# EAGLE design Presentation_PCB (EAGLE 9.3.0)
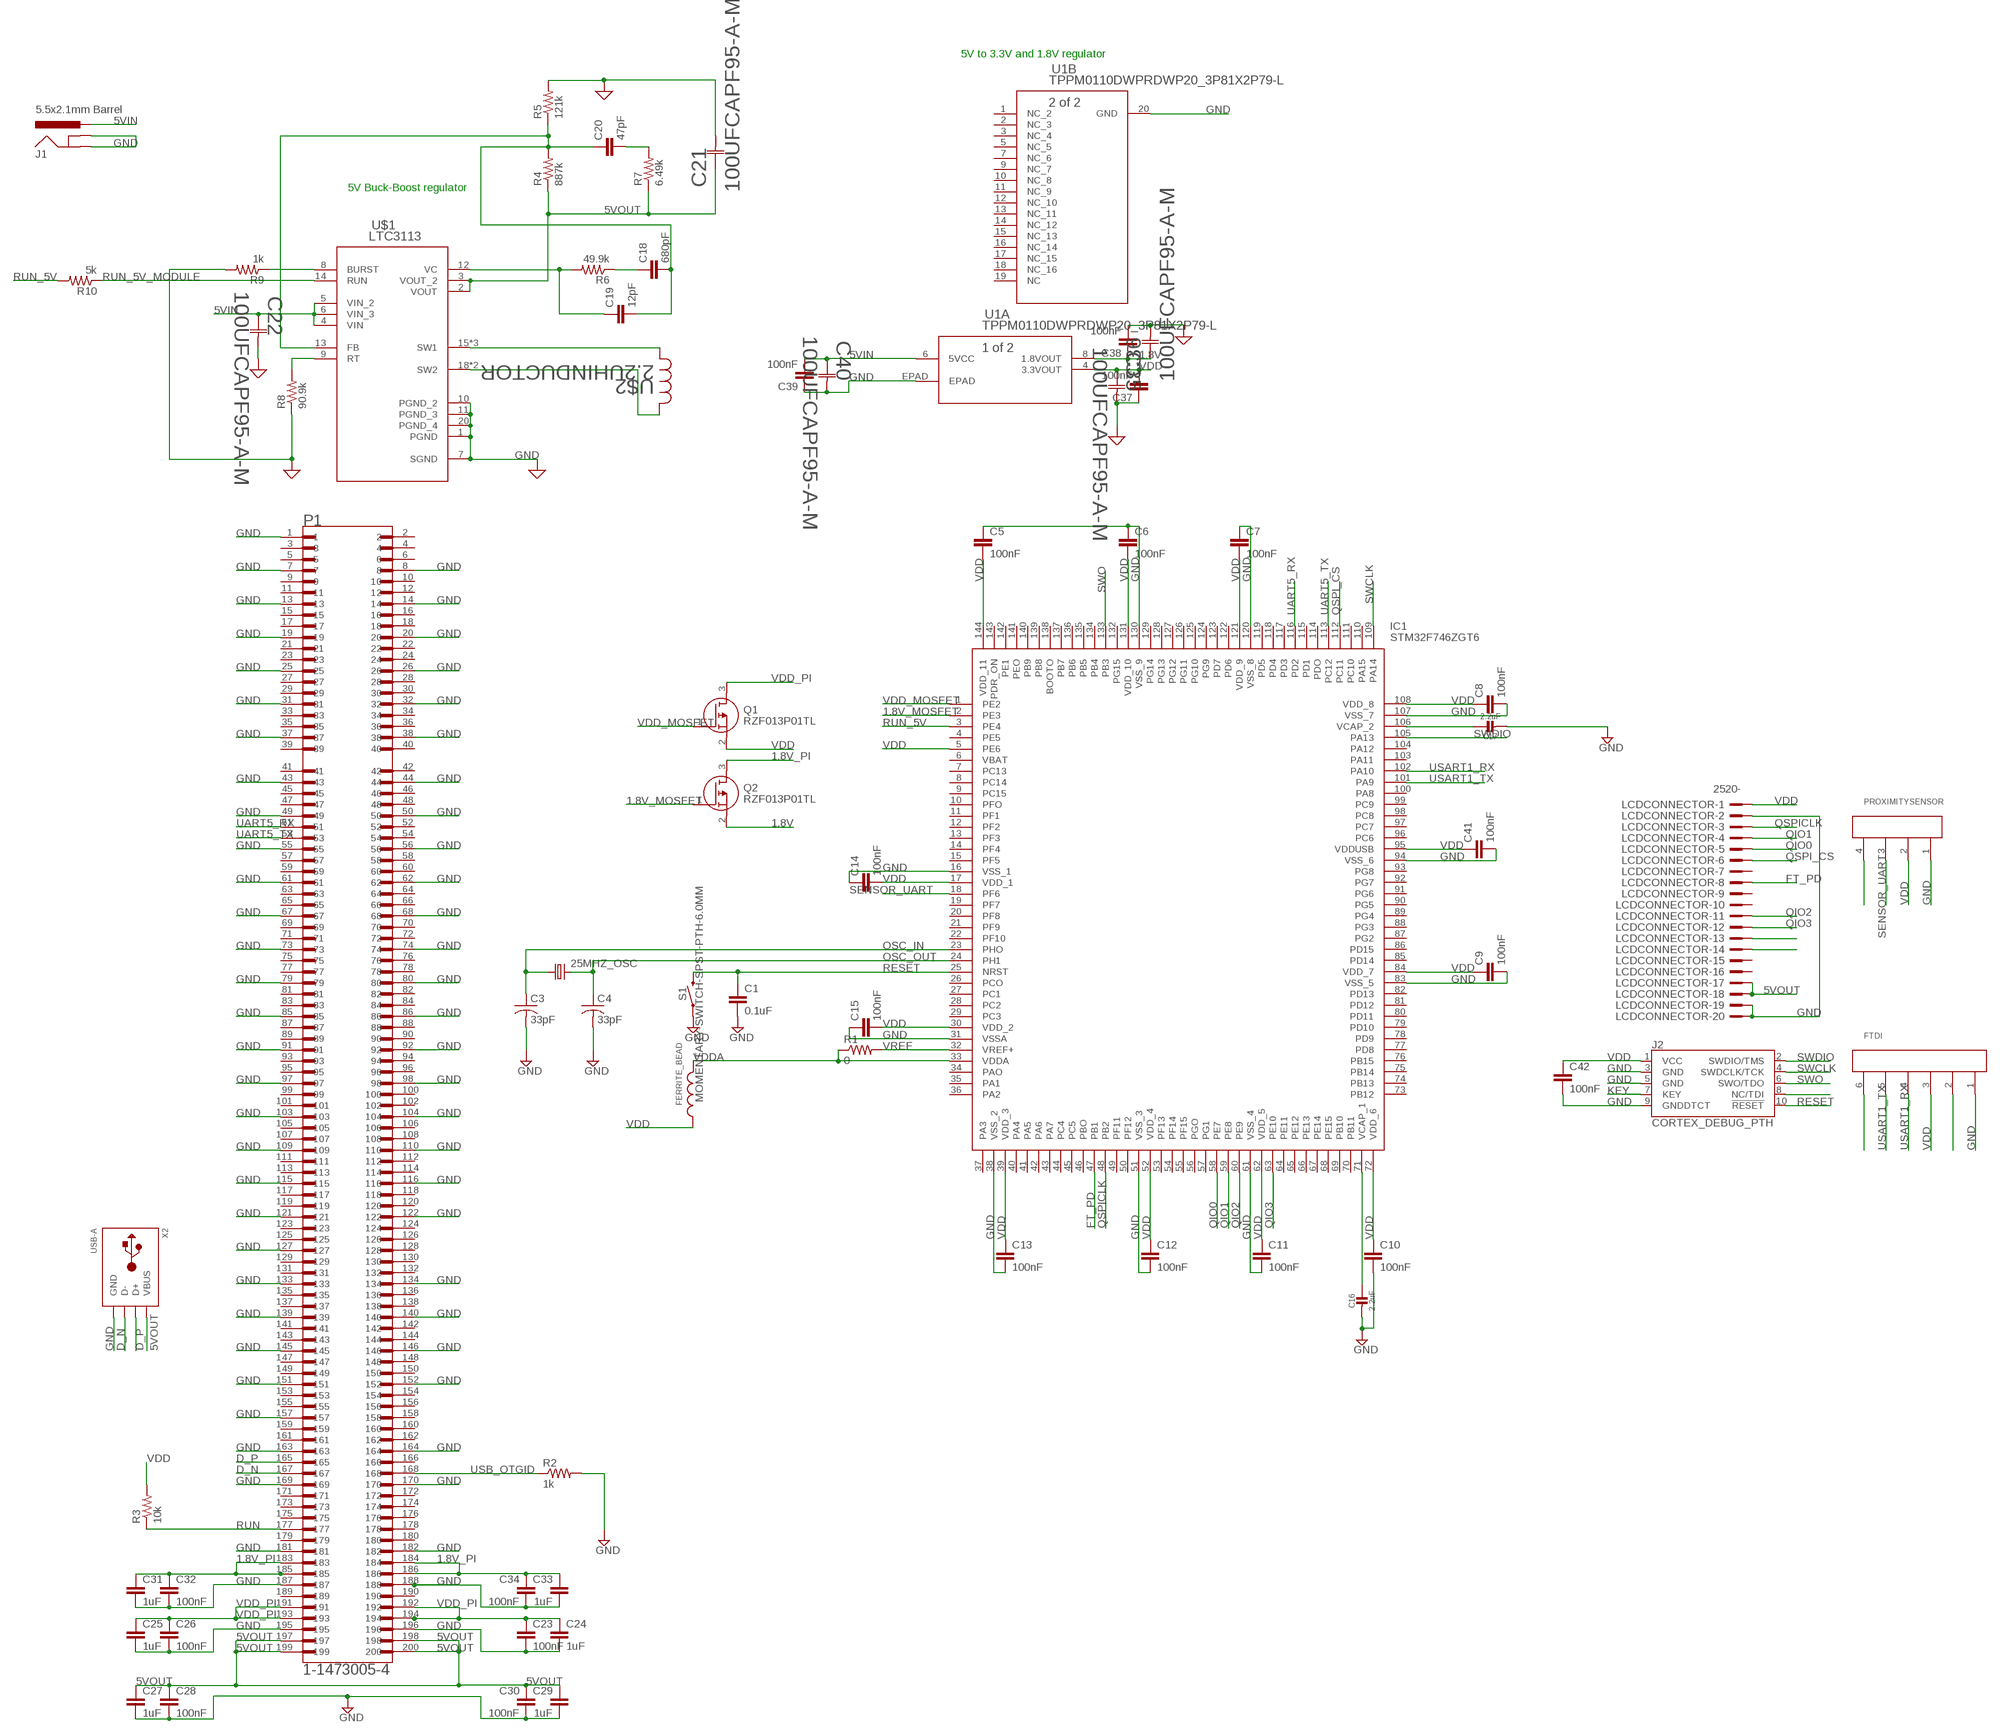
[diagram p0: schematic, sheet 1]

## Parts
25MHZ_OSC  CRYSTALHC49UP  [HC49UP]
C1  0.1uF  C-EUC0805  [C0805]
C3  33pF  C-USC0805  [C0805]
C4  33pF  C-USC0805  [C0805]
C5  100nF  C-EUC0805  [C0805]
C6  100nF  C-EUC0805  [C0805]
C7  100nF  C-EUC0805  [C0805]
C8  100nF  C-EUC0805  [C0805]
C9  100nF  C-EUC0805  [C0805]
C10  100nF  C-EUC0805  [C0805]
C11  100nF  C-EUC0805  [C0805]
C12  100nF  C-EUC0805  [C0805]
C13  100nF  C-EUC0805  [C0805]
C14  100nF  C-EUC0805  [C0805]
C15  100nF  C-EUC0805  [C0805]
C16  2.2uF  CAP_CERAMIC0805-NOOUTLINE  [0805-NO]
C17  2.2uF  CAP_CERAMIC0805-NOOUTLINE  [0805-NO]
C18  680pF  C-EUC0805  [C0805]
C19  12pF  C-EUC0805  [C0805]
C20  47pF  C-EUC0805  [C0805]
C21  100UFCAPF95-A-M  [F95-A-M]
C22  100UFCAPF95-A-M  [F95-A-M]
C23  100nF  C-EUC0805  [C0805]
C24  1uF  C-EUC0805  [C0805]
C25  1uF  C-EUC0805  [C0805]
C26  100nF  C-EUC0805  [C0805]
C27  1uF  C-EUC0805  [C0805]
C28  100nF  C-EUC0805  [C0805]
C29  1uF  C-EUC0805  [C0805]
C30  100nF  C-EUC0805  [C0805]
C31  1uF  C-EUC0805  [C0805]
C32  100nF  C-EUC0805  [C0805]
C33  1uF  C-EUC0805  [C0805]
C34  100nF  C-EUC0805  [C0805]
C35  100UFCAPF95-A-M  [F95-A-M]
C36  100UFCAPF95-A-M  [F95-A-M]
C37  100nF  C-EUC0805  [C0805]
C38  100nF  C-EUC0805  [C0805]
C39  100nF  C-EUC0805  [C0805]
C40  100UFCAPF95-A-M  [F95-A-M]
C41  100nF  C-EUC0805  [C0805]
C42  100nF  C-EUC0805  [C0805]
FERRITE_BEAD  WE-CBA_0805_782853112_HC  [WE-CBA_0805(W=4)]
FTDI  66100611622  [66100611622]
IC1  STM32F746ZGT6  [QFP50P2200X2200X160-144N]
J1  5.5x2.1mm Barrel  POWER_JACKSMD  [POWER_JACK_SMD]
J2  CORTEX_DEBUG_PTH  [2X5-PTH-1.27MM]
LCDCONNECTOR  2520-  [PAK100/2500-20]
P1  1-1473005-4  [TE_1-1473005-4]
PROXIMITYSENSOR  66100411622  [66100411622]
Q1  RZF013P01TL  [SOT65P210X85-3N]
Q2  RZF013P01TL  [SOT65P210X85-3N]
R1  0  R-US_R0805  [R0805]
R2  1k  R-US_R0805  [R0805]
R3  10k  R-US_R0805  [R0805]
R4  887k  R-US_R0805  [R0805]
R5  121k  R-US_R0805  [R0805]
R6  49.9k  R-US_R0805  [R0805]
R7  6.49k  R-US_R0805  [R0805]
R8  90.9k  R-US_R0805  [R0805]
R9  1k  R-US_R0805  [R0805]
R10  5k  R-US_R0805  [R0805]
S1  MOMENTARY-SWITCH-SPST-PTH-6.0MM  [TACTILE_SWITCH_PTH_6.0MM]
U1  TPPM0110DWPRDWP20_3P81X2P79-L  [DWP20_3P81X2P79-L]
U$1  LTC3113  [TSSOP-20_FE/CA]
U$2  2.2UHINDUCTOR  [IND_10040]
X2  USB-A  [MOLEX_480371000]

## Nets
1.8V: C36.1 C38.1 Q2.2(S) U1.8(A:1.8VOUT)
1.8V_MOSFET: IC1.2(PE3) Q2.1(G)
1.8V_PI: C31.1 C32.1 C33.1 C34.1 P1.183 P1.184 P1.185 P1.186 Q2.3(D)
5VIN: C22.1 C39.2 C40.1 J1.VIN0(PWR) U1.6(A:5VCC) U$1.4(VIN) U$1.5(VIN_2) U$1.6(VIN_3)
5VOUT: C21.1 C27.1 C28.1 C29.1 C30.1 LCDCONNECTOR.17 LCDCONNECTOR.18 P1.197 P1.198 P1.199 P1.200 R4.1 R7.1 U$1.2(VOUT) U$1.3(VOUT_2) X2.1(VBUS)
D_N [D]: P1.167 X2.2(D-)
D_P [D]: P1.165 X2.3(D+)
FT_PD: IC1.47(PB1) LCDCONNECTOR.8
GND: C1.2 C3.2 C4.2 C5.1 C6.1 C7.1 C8.2 C9.2 C10.2 C11.2 C12.2 C13.2 C14.1 C15.1 C16.2 C17.2 C21.2 C22.2 C23.2 C24.2 C25.2 C26.2 C27.2 C28.2 C29.2 C30.2 C31.2 C32.2 C33.2 C34.2 C35.2 C36.2 C37.1 C38.2 C39.1 C40.2 C41.2 C42.2 FTDI.1 IC1.16(VSS_1) IC1.31(VSSA) IC1.38(VSS_2) IC1.51(VSS_3) IC1.61(VSS_4) IC1.83(VSS_5) IC1.94(VSS_6) IC1.107(VSS_7) IC1.120(VSS_8) IC1.130(VSS_9) J1.GND(GNDBREAK) J1.P$4(GND) J2.3(GND) J2.5(GND) J2.9(GNDDTCT) LCDCONNECTOR.2 LCDCONNECTOR.19 LCDCONNECTOR.20 P1.1 P1.7 P1.8 P1.13 P1.14 P1.19 P1.20 P1.25 P1.26 P1.31 P1.32 P1.37 P1.38 P1.43 P1.44 P1.49 P1.50 P1.55 P1.56 P1.61 P1.62 P1.67 P1.68 P1.73 P1.74 P1.79 P1.80 P1.85 P1.86 P1.91 P1.92 P1.97 P1.98 P1.103 P1.104 P1.109 P1.110 P1.115 P1.116 P1.121 P1.122 P1.127 P1.133 P1.134 P1.139 P1.140 P1.145 P1.146 P1.151 P1.152 P1.157 P1.163 P1.164 P1.169 P1.170 P1.181 P1.182 P1.187 P1.188 P1.195 P1.196 PROXIMITYSENSOR.1 R2.2 R5.2 R8.1 R9.2 S1.1 U1.20(B:GND) U1.EPAD(A:EPAD) U$1.1(PGND) U$1.7(SGND) U$1.10(PGND_2) U$1.11(PGND_3) U$1.20(PGND_4) X2.4(GND) ; supply symbol labelled SUP
KEY: J2.7(KEY)
N$1: C16.1 IC1.71(VCAP_1)
N$2: C17.1 IC1.106(VCAP_2)
N$3: C20.2 R7.2
N$4: C19.1 R6.2 U$1.12(VC)
N$5: C18.1 R6.1
N$6: C18.2 C19.2 C20.1 R4.2 R5.1 U$1.13(FB)
N$7: U$1.15(SW1) U$1.16(SW1) U$1.17(SW1) U$2.2
N$8: U$1.18(SW2) U$1.19(SW2) U$2.1
N$9: R8.2 U$1.9(RT)
N$10: R9.1 U$1.8(BURST)
N$12: FTDI.2
N$15: PROXIMITYSENSOR.4
N$16: FTDI.6
N$19: J2.8(NC/TDI)
N$20: LCDCONNECTOR.13
N$21: LCDCONNECTOR.14
OSC_IN: 25MHZ_OSC.1 C3.1 IC1.23(PHO)
OSC_OUT: 25MHZ_OSC.2 C4.1 IC1.24(PH1)
QIO0: IC1.58(PE7) LCDCONNECTOR.5
QIO1: IC1.59(PE8) LCDCONNECTOR.4
QIO2: IC1.60(PE9) LCDCONNECTOR.11
QIO3: IC1.63(PE10) LCDCONNECTOR.12
QSPI_CS: IC1.112(PC11) LCDCONNECTOR.6
QSPICLK: IC1.48(PB2) LCDCONNECTOR.3
RESET: C1.1 IC1.25(NRST) J2.10(!RESET) S1.3
RUN: P1.177 R3.1
RUN_5V: IC1.3(PE4) R10.2
RUN_5V_MODULE: R10.1 U$1.14(RUN)
SENSOR_UART: IC1.18(PF6) PROXIMITYSENSOR.3
SWCLK: IC1.109(PA14) J2.4(SWDCLK/TCK)
SWDIO: IC1.105(PA13) J2.2(SWDIO/TMS)
SWO: IC1.133(PB3) J2.6(SWO/TDO)
UART5_RX: IC1.116(PD2) P1.51
UART5_TX: IC1.113(PC12) P1.53
USART1_RX: FTDI.4 IC1.102(PA10)
USART1_TX: FTDI.5 IC1.101(PA9)
USB_OTGID: P1.168 R2.1
VDD: C5.2 C6.2 C7.2 C8.1 C9.1 C10.1 C11.1 C12.1 C13.1 C14.2 C15.2 C35.1 C37.2 C41.1 C42.1 FERRITE_BEAD.1 FTDI.3 IC1.5(PE6) IC1.17(VDD_1) IC1.30(VDD_2) IC1.39(VDD_3) IC1.52(VDD_4) IC1.62(VDD_5) IC1.72(VDD_6) IC1.84(VDD_7) IC1.95(VDDUSB) IC1.108(VDD_8) IC1.121(VDD_9) IC1.131(VDD_10) IC1.144(VDD_11) J2.1(VCC) LCDCONNECTOR.1 PROXIMITYSENSOR.2 Q1.2(S) R3.2 U1.4(A:3.3VOUT)
VDD_MOSFET: IC1.1(PE2) Q1.1(G)
VDD_PI: C23.1 C24.1 C25.1 C26.1 P1.191 P1.192 P1.193 P1.194 Q1.3(D)
VDDA: FERRITE_BEAD.2 IC1.33(VDDA) R1.1
VREF: IC1.32(VREF+) R1.2
Unconnected: IC1.4(PE5) IC1.6(VBAT) IC1.7(PC13) IC1.8(PC14) IC1.9(PC15) IC1.10(PFO) IC1.11(PF1) IC1.12(PF2) IC1.13(PF3) IC1.14(PF4) IC1.15(PF5) IC1.19(PF7) IC1.20(PF8) IC1.21(PF9) IC1.22(PF10) IC1.26(PCO) IC1.27(PC1) IC1.28(PC2) IC1.29(PC3) IC1.34(PAO) IC1.35(PA1) IC1.36(PA2) IC1.37(PA3) IC1.40(PA4) IC1.41(PA5) IC1.42(PA6) IC1.43(PA7) IC1.44(PC4) IC1.45(PC5) IC1.46(PBO) IC1.49(PF11) IC1.50(PF12) IC1.53(PF13) IC1.54(PF14) IC1.55(PF15) IC1.56(PGO) IC1.57(PG1) IC1.64(PE11) IC1.65(PE12) IC1.66(PE13) IC1.67(PE14) IC1.68(PE15) IC1.69(PB10) IC1.70(PB11) IC1.73(PB12) IC1.74(PB13) IC1.75(PB14) IC1.76(PB15) IC1.77(PD8) IC1.78(PD9) IC1.79(PD10) IC1.80(PD11) IC1.81(PD12) IC1.82(PD13) IC1.85(PD14) IC1.86(PD15) IC1.87(PG2) IC1.88(PG3) IC1.89(PG4) IC1.90(PG5) IC1.91(PG6) IC1.92(PG7) IC1.93(PG8) IC1.96(PC6) IC1.97(PC7) IC1.98(PC8) IC1.99(PC9) IC1.100(PA8) IC1.103(PA11) IC1.104(PA12) IC1.110(PA15) IC1.111(PC10) IC1.114(PDO) IC1.115(PD1) IC1.117(PD3) IC1.118(PD4) IC1.119(PD5) IC1.122(PD6) IC1.123(PD7) IC1.124(PG9) IC1.125(PG10) IC1.126(PG11) IC1.127(PG12) IC1.128(PG13) IC1.129(PG14) IC1.132(PG15) IC1.134(PB4) IC1.135(PB5) IC1.136(PB6) IC1.137(PB7) IC1.138(BOOTO) IC1.139(PB8) IC1.140(PB9) IC1.141(PEO) IC1.142(PE1) IC1.143(PDR_ON) LCDCONNECTOR.7 LCDCONNECTOR.9 LCDCONNECTOR.10 LCDCONNECTOR.15 LCDCONNECTOR.16 P1.2 P1.3 P1.4 P1.5 P1.6 P1.9 P1.10 P1.11 P1.12 P1.15 P1.16 P1.17 P1.18 P1.21 P1.22 P1.23 P1.24 P1.27 P1.28 P1.29 P1.30 P1.33 P1.34 P1.35 P1.36 P1.39 P1.40 P1.41 P1.42 P1.45 P1.46 P1.47 P1.48 P1.52 P1.54 P1.57 P1.58 P1.59 P1.60 P1.63 P1.64 P1.65 P1.66 P1.69 P1.70 P1.71 P1.72 P1.75 P1.76 P1.77 P1.78 P1.81 P1.82 P1.83 P1.84 P1.87 P1.88 P1.89 P1.90 P1.93 P1.94 P1.95 P1.96 P1.99 P1.100 P1.101 P1.102 P1.105 P1.106 P1.107 P1.108 P1.111 P1.112 P1.113 P1.114 P1.117 P1.118 P1.119 P1.120 P1.123 P1.124 P1.125 P1.126 P1.128 P1.129 P1.130 P1.131 P1.132 P1.135 P1.136 P1.137 P1.138 P1.141 P1.142 P1.143 P1.144 P1.147 P1.148 P1.149 P1.150 P1.153 P1.154 P1.155 P1.156 P1.158 P1.159 P1.160 P1.161 P1.162 P1.166 P1.171 P1.172 P1.173 P1.174 P1.175 P1.176 P1.178 P1.179 P1.180 P1.189 P1.190 U1.1(B:NC_2) U1.2(B:NC_3) U1.3(B:NC_4) U1.5(B:NC_5) U1.7(B:NC_6) U1.9(B:NC_7) U1.10(B:NC_8) U1.11(B:NC_9) U1.12(B:NC_10) U1.13(B:NC_11) U1.14(B:NC_12) U1.15(B:NC_13) U1.16(B:NC_14) U1.17(B:NC_15) U1.18(B:NC_16) U1.19(B:NC)

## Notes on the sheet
- 5V to 3.3V and 1.8V regulator
- 5V Buck-Boost regulator

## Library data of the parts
25MHZ_OSC = adafruit:CRYSTAL: CRYSTAL; OC_FARNELL: unknown; OC_NEWARK: unknown
C1 C5-C15 C18-C20 C23-C34 C37-C39 C41 C42 = rcl:C-EU: CAPACITOR, European symbol; SPICEPREFIX: C
C3 C4 = adafruit:C-US: CAPACITOR, American symbol
C16 C17 = audio amplifier example:CAP_CERAMIC
C21 C22 C35 C36 C40 = 477_LIBRARY:100UFCAP; MANUFACTURER_PART_NUMBER: F951A107KAAAQ2; VENDOR: AVX Corporation
FERRITE_BEAD = Wurth_Elektronik_Passive_rev18f:WE-CBA_0805: WE-CBA SMD EMI Suppression Ferrite Bead
FTDI = Wurth_Elektronik_Electromechanic_Wire_to_Board_Connectors_rev18a:66100611622: WIRE TO BOARD CONNECTION - 2.54 MM - SHROUDED HEADER - STRAIGHT - GLOW WIRE PLASTIC - WR-WTB =>ConWTB254 661006116222 Characteristics INSULATOR: PA46G15 FLAMMABILITY RATING: UL94V0 COLOR: BLACK METAL: PHOSPHOR BRONZE PLATING: TIN OVER Ni QUALITY CLASS: 25 MATING CYCLES OPERATING TEMPERATURE:-40°C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
IC1 = 477_LIBRARY:STM32F746ZGT6: ARM Microcontrollers - MCU High-performance and DSP with FPU, ARM Cortex-M7 MCU with 1 Mbytes Flash, 200 MHz CPU, Art Accelerator, L1 cache, SDRAM Source: Datasheet; DESCRIPTION: ARM Microcontrollers - MCU High-performance and DSP with FPU, ARM Cortex-M7 MCU with 1 Mbytes Flash, 200 MHz CPU, Art Accelerator, L1 cache, SDRAM; HEIGHT: 1.6mm; MANUFACTURER_NAME: STMicroelectronics; MANUFACTURER_PART_NUMBER: STM32F746ZGT6; MOUSER_PART_NUMBER: 511-STM32F746ZGT6; MOUSER_PRICE-STOCK: https://www.mouser.com/Search/Refine.aspx?Keyword=511-STM32F746ZGT6; RS_PART_NUMBER: 8820290; RS_PRICE-STOCK: http://uk.rs-online.com/web/p/products/8820290
J1 = SparkFun-Connectors:POWER_JACK: Power Jack Connector This is the standard 5.5mm barrel jack for power. The PTH is the most common, proven, reliable, footprint. The Slot footprint only works if the mill layer is transmitted to the PCB fab house so be warned. Here are the connectors we sell at SparkFun: DC Barrel Power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; PROD_ID: CONN-08106; SF_ID: PRT-12748
J2 = SparkFun-Connectors:CORTEX_DEBUG: Cortex Debug Connector - 10 pin Supports JTAG debug, Serial Wire debug, and Serial Wire Viewer. PTH and SMD connector options available. General Connector Information Products: PTH Connector -via Digi-Key SparkFun PSoc SparkFun T
LCDCONNECTOR = con-3m:2520-: 3M (TM) Pak 100 4-Wall Header Source: 3M; OC_FARNELL: unknown; OC_NEWARK: unknown
P1 = Rpi-DDR2:1-1473005-4: Conn SO DIMM Socket SKT 200 POS 0.6mm Solder RA SMD Tray; AVAILABILITY: Unavailable; CENTERLINE_PITCH: .6 mm[.024 in]; COMMENT: 1-1473005-4; DESCRIPTION: SEMI-HARD TRAY DDR2 SODIMM SOCKET 200P 5; MF: TE Connectivity; MP: 1-1473005-4; NUMBER_OF_POSITIONS: 200; PACKAGE: None; PRICE: None; PRODUCT_TYPE: Socket; TE_PURCHASE_URL: https://www.te.com/usa-en/product-1-1473005-4.html?te_bu=Cor&te_type=disp&te_campaign=seda_glo_cor-seda-global-disp-prtnr-fy19-seda-model-bom-cta_sma-317_1&elqCampaignId=32493
PROXIMITYSENSOR = Wurth_Elektronik_Electromechanic_Wire_to_Board_Connectors_rev18a:66100411622: WIRE TO BOARD CONNECTION - 2.54 MM - SHROUDED HEADER - STRAIGHT - GLOW WIRE PLASTIC - WR-WTB =>ConWTB254 661004116222 Characteristics INSULATOR: PA46G15 FLAMMABILITY RATING: UL94V0 COLOR: BLACK METAL: PHOSPHOR BRONZE PLATING: TIN OVER Ni QUALITY CLASS: 25 MATING CYCLES OPERATING TEMPERATURE:-40°C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
Q1 Q2 = Pchannel:RZF013P01TL: 1.5V Drive Pch MOSFET: MOSFETs are made as ultra-low ON-resistance by the micro-processing technologies suitable for mobilr equipment for low current consumption. In wide lineup including compact type, high-power type and complex type to meet in the market. Source: Datasheet; DESCRIPTION: 1.5V Drive Pch MOSFET: MOSFETs are made as ultra-low ON-resistance by the micro-processing technologies suitable for mobilr equipment for low current consumption. In wide lineup including compact type, high-power type and complex type to meet in the market.; HEIGHT: 0.85mm; MANUFACTURER_NAME: ROHM Semiconductor; MANUFACTURER_PART_NUMBER: RZF013P01TL; MOUSER_PART_NUMBER: 755-RZF013P01TL; MOUSER_PRICE-STOCK: https://www.mouser.com/Search/Refine.aspx?Keyword=755-RZF013P01TL
R1-R3 = audio amplifier example:R-US_: RESISTOR, American symbol
R4-R10 = resistor:R-US_: RESISTOR, American symbol
S1 = SparkFun-Switches:MOMENTARY-SWITCH-SPST: Momentary Switch (Pushbutton) - SPST; PROD_ID: SWCH-08441; SF_SKU: COM-00097
U1 = 477_LIBRARY:TPPM0110DWPR; MANUFACTURER_PART_NUMBER: TPPM0110DWPR; VENDOR: Texas Instruments
U$1 = 477_LIBRARY:LTC3113
U$2 = 477_LIBRARY:2.2UHINDUCTOR
X2 = adafruit:USB-A: USB type A 'plug' Used for things that can directly connect to a USB port, say USB key

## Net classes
1 D: width 0.203 mm

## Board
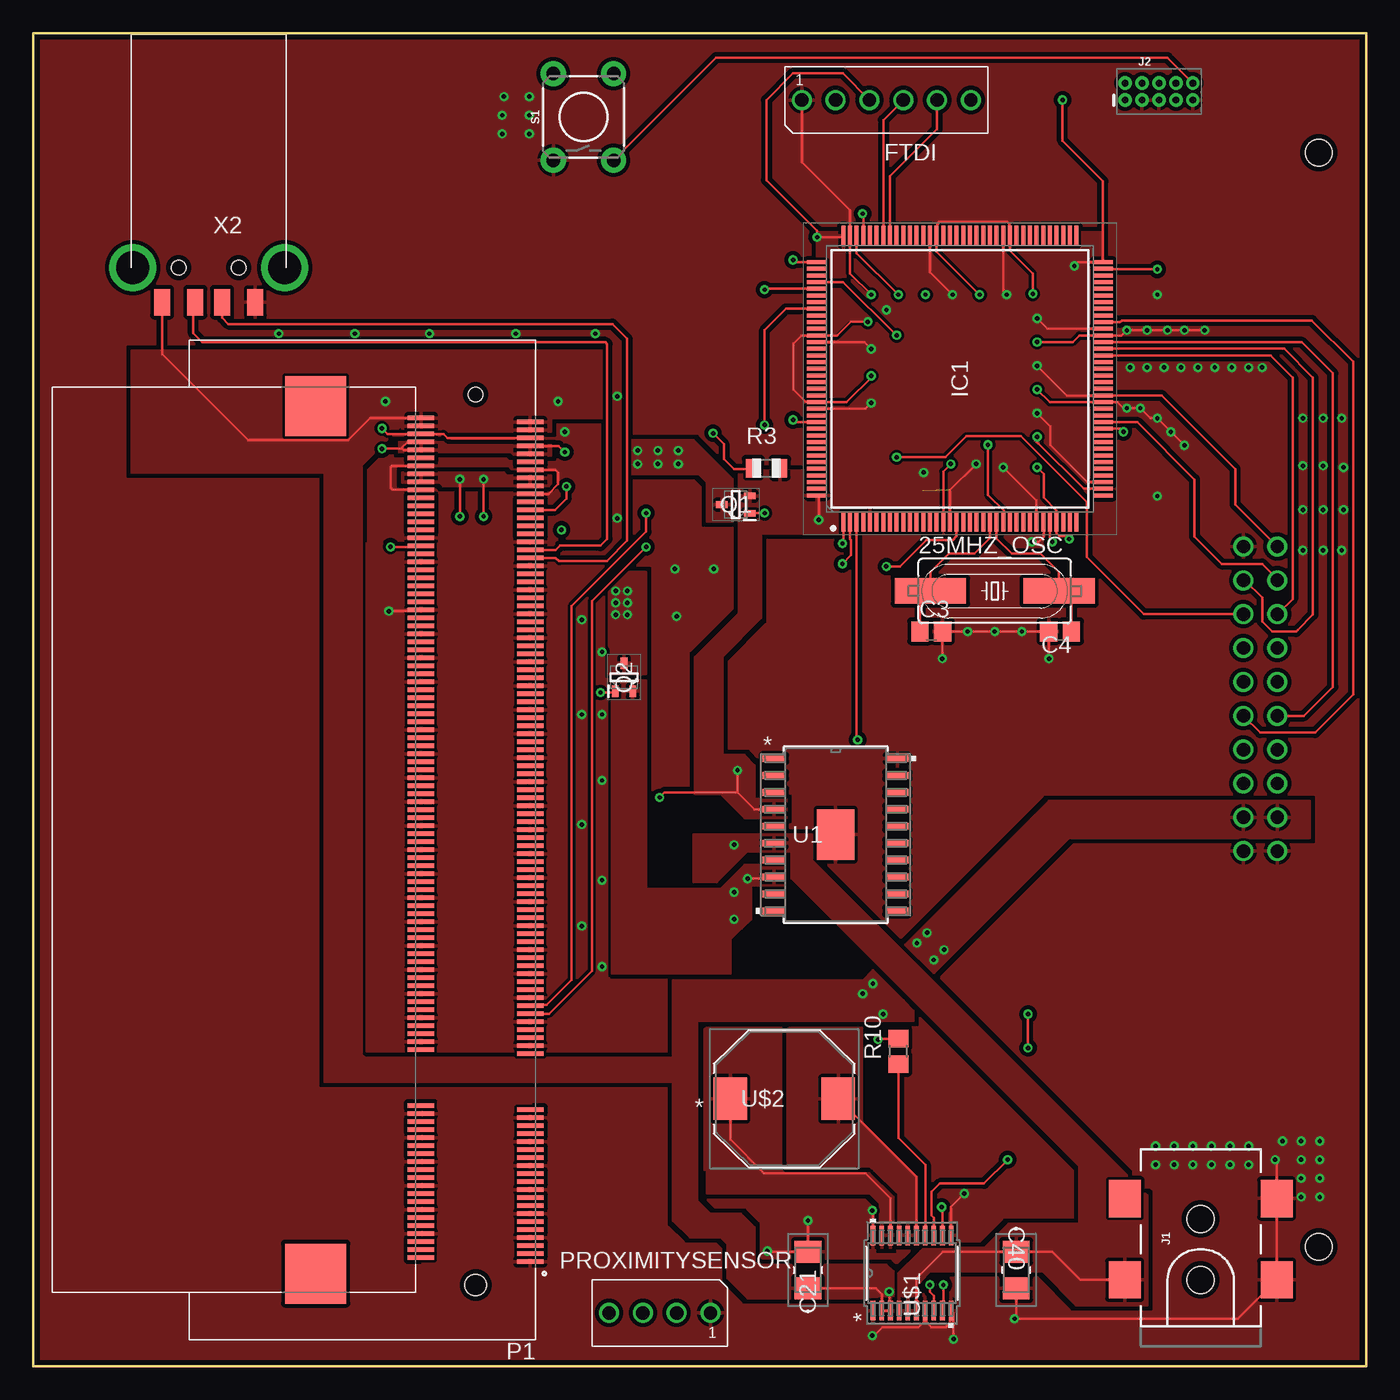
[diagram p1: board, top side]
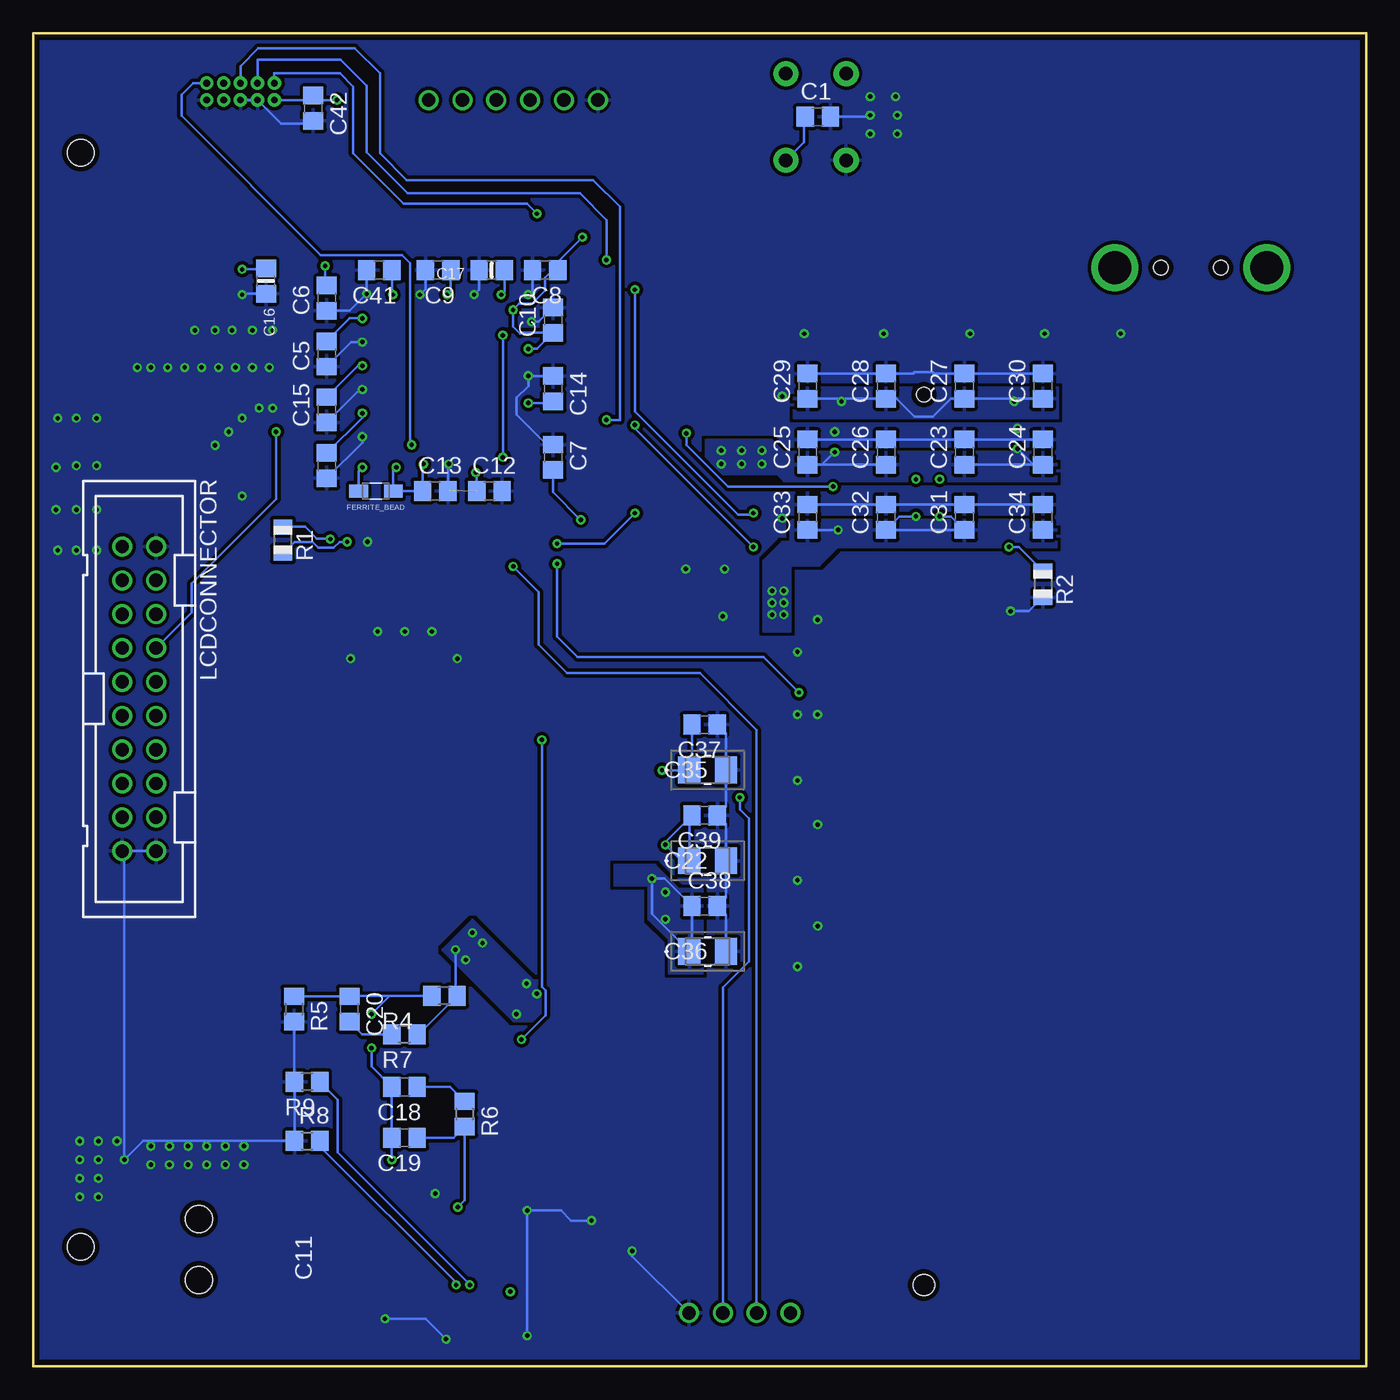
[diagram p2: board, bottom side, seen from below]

Size 100 x 100 mm. Coordinates in mm from the lower left corner, seen from the top.
Outline: 0,0 100,0 100,100 0,100 0,0
Copper layers (1*16): Top 0.0356mm / dielectric 1.5011mm / Bottom 0.0356mm
Design rules "ECE_Senior_Design": minimum track width 8mil, minimum drill 13mil, track to track 8mil, track to pad 8mil, pad to pad 6mil, via to via 8mil, smd to smd 6mil, copper to edge 15mil, drill to drill 8mil, minimum pad ring 7mil, minimum via ring 7mil, stop-mask expansion 3mil, vias tented up to drill 0mil, thermal gap 10mil
Holes 2 mm at 96.45,8.95 96.45,91.05

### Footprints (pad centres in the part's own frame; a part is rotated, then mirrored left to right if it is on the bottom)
HC49UP = smd 5.334 x 1.93: 1 -4.826,0; 2 4.826,0
C0805 = smd 1.3 x 1.5: 1 -0.95,0; 2 0.95,0
C0805' = smd 1.3 x 1.5: 1 -0.85,0; 2 0.85,0
0805-NO = smd 1.3 x 1.5: 1 -0.95,0; 2 0.95,0
F95-A-M = smd 1.651 x 2.007: 1 -1.384,0; 2 1.384,0
WE-CBA_0805(W=4) = smd 1.4 x 1: 1 -1.3,0; 2 1.3,0
66100611622 = drill 1: 1 6.35,0; 2 3.81,0; 3 1.27,0; 4 -1.27,0; 5 -3.81,0; 6 -6.35,0
QFP50P2200X2200X160-144N = smd 1.475 x 0.3: 1 -10.738,8.75; 2 -10.738,8.25; 3 -10.738,7.75; 4 -10.738,7.25; 5 -10.738,6.75; 6 -10.738,6.25; 7 -10.738,5.75; 8 -10.738,5.25; 9 -10.738,4.75; 10 -10.738,4.25; 11 -10.738,3.75; 12 -10.738,3.25; 13 -10.738,2.75; 14 -10.738,2.25; 15 -10.738,1.75; 16 -10.738,1.25; 17 -10.738,0.75; 18 -10.738,0.25; 19 -10.738,-0.25; 20 -10.738,-0.75; 21 -10.738,-1.25; 22 -10.738,-1.75; 23 -10.738,-2.25; 24 -10.738,-2.75; 25 -10.738,-3.25; 26 -10.738,-3.75; 27 -10.738,-4.25; 28 -10.738,-4.75; 29 -10.738,-5.25; 30 -10.738,-5.75; 31 -10.738,-6.25; 32 -10.738,-6.75; 33 -10.738,-7.25; 34 -10.738,-7.75; 35 -10.738,-8.25; 36 -10.738,-8.75; 73 10.738,-8.75; 74 10.738,-8.25; 75 10.738,-7.75; 76 10.738,-7.25; 77 10.738,-6.75; 78 10.738,-6.25; 79 10.738,-5.75; 80 10.738,-5.25; 81 10.738,-4.75; 82 10.738,-4.25; 83 10.738,-3.75; 84 10.738,-3.25; 85 10.738,-2.75; 86 10.738,-2.25; 87 10.738,-1.75; 88 10.738,-1.25; 89 10.738,-0.75; 90 10.738,-0.25; 91 10.738,0.25; 92 10.738,0.75; 93 10.738,1.25; 94 10.738,1.75; 95 10.738,2.25; 96 10.738,2.75; 97 10.738,3.25; 98 10.738,3.75; 99 10.738,4.25; 100 10.738,4.75; 101 10.738,5.25; 102 10.738,5.75; 103 10.738,6.25; 104 10.738,6.75; 105 10.738,7.25; 106 10.738,7.75; 107 10.738,8.25; 108 10.738,8.75 | smd 0.3 x 1.475: 37 -8.75,-10.738; 38 -8.25,-10.738; 39 -7.75,-10.738; 40 -7.25,-10.738; 41 -6.75,-10.738; 42 -6.25,-10.738; 43 -5.75,-10.738; 44 -5.25,-10.738; 45 -4.75,-10.738; 46 -4.25,-10.738; 47 -3.75,-10.738; 48 -3.25,-10.738; 49 -2.75,-10.738; 50 -2.25,-10.738; 51 -1.75,-10.738; 52 -1.25,-10.738; 53 -0.75,-10.738; 54 -0.25,-10.738; 55 0.25,-10.738; 56 0.75,-10.738; 57 1.25,-10.738; 58 1.75,-10.738; 59 2.25,-10.738; 60 2.75,-10.738; 61 3.25,-10.738; 62 3.75,-10.738; 63 4.25,-10.738; 64 4.75,-10.738; 65 5.25,-10.738; 66 5.75,-10.738; 67 6.25,-10.738; 68 6.75,-10.738; 69 7.25,-10.738; 70 7.75,-10.738; 71 8.25,-10.738; 72 8.75,-10.738; 109 8.75,10.738; 110 8.25,10.738; 111 7.75,10.738; 112 7.25,10.738; 113 6.75,10.738; 114 6.25,10.738; 115 5.75,10.738; 116 5.25,10.738; 117 4.75,10.738; 118 4.25,10.738; 119 3.75,10.738; 120 3.25,10.738; 121 2.75,10.738; 122 2.25,10.738; 123 1.75,10.738; 124 1.25,10.738; 125 0.75,10.738; 126 0.25,10.738; 127 -0.25,10.738; 128 -0.75,10.738; 129 -1.25,10.738; 130 -1.75,10.738; 131 -2.25,10.738; 132 -2.75,10.738; 133 -3.25,10.738; 134 -3.75,10.738; 135 -4.25,10.738; 136 -4.75,10.738; 137 -5.25,10.738; 138 -5.75,10.738; 139 -6.25,10.738; 140 -6.75,10.738; 141 -7.25,10.738; 142 -7.75,10.738; 143 -8.25,10.738; 144 -8.75,10.738
POWER_JACK_SMD = smd 2.8 x 2.4: GND 0,-5.7; P$4 6.1,-5.7; VIN0 0,5.7; VIN1 6.1,5.7 | hole 2.032: 0,0; 4.572,0
2X5-PTH-1.27MM = drill 0.508 pad 1: 1 -2.54,-0.635; 2 -2.54,0.635; 3 -1.27,-0.635; 4 -1.27,0.635; 5 0,-0.635; 6 0,0.635; 7 1.27,-0.635; 8 1.27,0.635; 9 2.54,-0.635; 10 2.54,0.635
PAK100/2500-20 = drill 1 pad 1.422: 1 -11.43,-1.27; 2 -11.43,1.27; 3 -8.89,-1.27; 4 -8.89,1.27; 5 -6.35,-1.27; 6 -6.35,1.27; 7 -3.81,-1.27; 8 -3.81,1.27; 9 -1.27,-1.27; 10 -1.27,1.27; 11 1.27,-1.27; 12 1.27,1.27; 13 3.81,-1.27; 14 3.81,1.27; 15 6.35,-1.27; 16 6.35,1.27; 17 8.89,-1.27; 18 8.89,1.27; 19 11.43,-1.27; 20 11.43,1.27
TE_1-1473005-4 = smd 2 x 0.35: 1 -4.1,31.65; 2 4.1,31.35; 3 -4.1,31.05; 4 4.1,30.75; 5 -4.1,30.45; 6 4.1,30.15; 7 -4.1,29.85; 8 4.1,29.55; 9 -4.1,29.25; 10 4.1,28.95; 11 -4.1,28.65; 12 4.1,28.35; 13 -4.1,28.05; 14 4.1,27.75; 15 -4.1,27.45; 16 4.1,27.15; 17 -4.1,26.85; 18 4.1,26.55; 19 -4.1,26.25; 20 4.1,25.95; 21 -4.1,25.65; 22 4.1,25.35; 23 -4.1,25.05; 24 4.1,24.75; 25 -4.1,24.45; 26 4.1,24.15; 27 -4.1,23.85; 28 4.1,23.55; 29 -4.1,23.25; 30 4.1,22.95; 31 -4.1,22.65; 32 4.1,22.35; 33 -4.1,22.05; 34 4.1,21.75; 35 -4.1,21.45; 36 4.1,21.15; 37 -4.1,20.85; 38 4.1,20.55; 39 -4.1,20.25; 40 4.1,19.95; 41 -4.1,16.05; 42 4.1,15.75; 43 -4.1,15.45; 44 4.1,15.15; 45 -4.1,14.85; 46 4.1,14.55; 47 -4.1,14.25; 48 4.1,13.95; 49 -4.1,13.65; 50 4.1,13.35; 51 -4.1,13.05; 52 4.1,12.75; 53 -4.1,12.45; 54 4.1,12.15; 55 -4.1,11.85; 56 4.1,11.55; 57 -4.1,11.25; 58 4.1,10.95; 59 -4.1,10.65; 60 4.1,10.35; 61 -4.1,10.05; 62 4.1,9.75; 63 -4.1,9.45; 64 4.1,9.15; 65 -4.1,8.85; 66 4.1,8.55; 67 -4.1,8.25; 68 4.1,7.95; 69 -4.1,7.65; 70 4.1,7.35; 71 -4.1,7.05; 72 4.1,6.75; 73 -4.1,6.45; 74 4.1,6.15; 75 -4.1,5.85; 76 4.1,5.55; 77 -4.1,5.25; 78 4.1,4.95; 79 -4.1,4.65; 80 4.1,4.35; 81 -4.1,4.05; 82 4.1,3.75; 83 -4.1,3.45; 84 4.1,3.15; 85 -4.1,2.85; 86 4.1,2.55; 87 -4.1,2.25; 88 4.1,1.95; 89 -4.1,1.65; 90 4.1,1.35; 91 -4.1,1.05; 92 4.1,0.75; 93 -4.1,0.45; 94 4.1,0.15; 95 -4.1,-0.15; 96 4.1,-0.45; 97 -4.1,-0.75; 98 4.1,-1.05; 99 -4.1,-1.35; 100 4.1,-1.65; 101 -4.1,-1.95; 102 4.1,-2.25; 103 -4.1,-2.55; 104 4.1,-2.85; 105 -4.1,-3.15; 106 4.1,-3.45; 107 -4.1,-3.75; 108 4.1,-4.05; 109 -4.1,-4.35; 110 4.1,-4.65; 111 -4.1,-4.95; 112 4.1,-5.25; 113 -4.1,-5.55; 114 4.1,-5.85; 115 -4.1,-6.15; 116 4.1,-6.45; 117 -4.1,-6.75; 118 4.1,-7.05; 119 -4.1,-7.35; 120 4.1,-7.65; 121 -4.1,-7.95; 122 4.1,-8.25; 123 -4.1,-8.55; 124 4.1,-8.85; 125 -4.1,-9.15; 126 4.1,-9.45; 127 -4.1,-9.75; 128 4.1,-10.05; 129 -4.1,-10.35; 130 4.1,-10.65; 131 -4.1,-10.95; 132 4.1,-11.25; 133 -4.1,-11.55; 134 4.1,-11.85; 135 -4.1,-12.15; 136 4.1,-12.45; 137 -4.1,-12.75; 138 4.1,-13.05; 139 -4.1,-13.35; 140 4.1,-13.65; 141 -4.1,-13.95; 142 4.1,-14.25; 143 -4.1,-14.55; 144 4.1,-14.85; 145 -4.1,-15.15; 146 4.1,-15.45; 147 -4.1,-15.75; 148 4.1,-16.05; 149 -4.1,-16.35; 150 4.1,-16.65; 151 -4.1,-16.95; 152 4.1,-17.25; 153 -4.1,-17.55; 154 4.1,-17.85; 155 -4.1,-18.15; 156 4.1,-18.45; 157 -4.1,-18.75; 158 4.1,-19.05; 159 -4.1,-19.35; 160 4.1,-19.65; 161 -4.1,-19.95; 162 4.1,-20.25; 163 -4.1,-20.55; 164 4.1,-20.85; 165 -4.1,-21.15; 166 4.1,-21.45; 167 -4.1,-21.75; 168 4.1,-22.05; 169 -4.1,-22.35; 170 4.1,-22.65; 171 -4.1,-22.95; 172 4.1,-23.25; 173 -4.1,-23.55; 174 4.1,-23.85; 175 -4.1,-24.15; 176 4.1,-24.45; 177 -4.1,-24.75; 178 4.1,-25.05; 179 -4.1,-25.35; 180 4.1,-25.65; 181 -4.1,-25.95; 182 4.1,-26.25; 183 -4.1,-26.55; 184 4.1,-26.85; 185 -4.1,-27.15; 186 4.1,-27.45; 187 -4.1,-27.75; 188 4.1,-28.05; 189 -4.1,-28.35; 190 4.1,-28.65; 191 -4.1,-28.95; 192 4.1,-29.25; 193 -4.1,-29.55; 194 4.1,-29.85; 195 -4.1,-30.15; 196 4.1,-30.45; 197 -4.1,-30.75; 198 4.1,-31.05; 199 -4.1,-31.35; 200 4.1,-31.65 | smd 4.6 x 4.5: P1 12,32.55; P2 12,-32.55 | hole 1.6: 0,33.4 | hole 1.1: 0,-33.4
66100411622 = drill 1: 1 3.81,0; 2 1.27,0; 3 -1.27,0; 4 -3.81,0
SOT65P210X85-3N = smd 0.85 x 0.5: 1 -1.05,0.65; 2 -1.05,-0.65; 3 1.05,0
R0805 = smd 1.1 x 1.4: 1 -1,0; 2 1,0
R0805' = smd 1.3 x 1.5: 1 -0.95,0; 2 0.95,0
TACTILE_SWITCH_PTH_6.0MM = drill 1.016 pad 1.88: 1 -3.251,2.261; 2 3.251,2.261; 3 -3.251,-2.261; 4 3.251,-2.261
DWP20_3P81X2P79-L = smd 1.676 x 0.508: 1 -4.636,5.715; 2 -4.636,4.445; 3 -4.636,3.175; 4 -4.636,1.905; 5 -4.636,0.635; 6 -4.636,-0.635; 7 -4.636,-1.905; 8 -4.636,-3.175; 9 -4.636,-4.445; 10 -4.636,-5.715; 11 4.636,-5.715; 12 4.636,-4.445; 13 4.636,-3.175; 14 4.636,-1.905; 15 4.636,-0.635; 16 4.636,0.635; 17 4.636,1.905; 18 4.636,3.175; 19 4.636,4.445; 20 4.636,5.715 | smd 2.79 x 3.81: EPAD 0,0
TSSOP-20_FE/CA = smd 1.473 x 0.356: 1 -2.819,2.926; 2 -2.819,2.276; 3 -2.819,1.626; 4 -2.819,0.975; 5 -2.819,0.325; 6 -2.819,-0.325; 7 -2.819,-0.975; 8 -2.819,-1.626; 9 -2.819,-2.276; 10 -2.819,-2.926; 11 2.819,-2.926; 12 2.819,-2.276; 13 2.819,-1.626; 14 2.819,-0.975; 15 2.819,-0.325; 16 2.819,0.325; 17 2.819,0.975; 18 2.819,1.626; 19 2.819,2.276; 20 2.819,2.926
IND_10040 = smd 2.5 x 3.2: 1 -4.05,0; 2 4.05,0
MOLEX_480371000 = smd 1.2 x 2: 1 3.5,2.6; 2 1,2.6; 3 -1,2.6; 4 -3.5,2.6 | drill 2.5: M1 -5.7,0; M2 5.7,0 | hole 1.1: -2.25,0; 2.25,0

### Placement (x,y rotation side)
25MHZ_OSC  72.14,58.17 0 top
C1  41.15,93.73 0 bottom
C3  33pF  [C0805']  67.37,55.13 0 top
C4  33pF  [C0805']  77.03,55.13 180 top
C5  77.98,75.95 90 bottom
C6  77.98,80.14 90 bottom
C7  61,68.2 270 bottom
C8  61.59,82.23 180 bottom
C9  69.63,82.23 180 bottom
C10  61,78.49 90 bottom
C11  77.98,67.56 270 bottom
C12  65.79,65.66 0 bottom
C13  69.84,65.66 0 bottom
C14  61,73.34 270 bottom
C15  77.98,71.75 90 bottom
C16  82.55,81.41 270 bottom
C17  65.61,82.23 180 bottom
C18  72.15,20.95 180 bottom
C19  72.15,17.14 180 bottom
C20  76.28,26.8 270 bottom
C21  58.12,7.21 90 top
C22  49.4,37.92 0 bottom
C23  30.14,68.58 90 bottom
C24  24.26,68.58 90 bottom
C25  41.91,68.58 90 bottom
C26  36.03,68.58 90 bottom
C27  30.14,73.53 90 bottom
C28  36.03,73.53 90 bottom
C29  41.91,73.53 90 bottom
C30  24.26,73.53 90 bottom
C31  30.14,63.69 90 bottom
C32  36.03,63.69 90 bottom
C33  41.91,63.69 90 bottom
C34  24.26,63.69 90 bottom
C35  49.4,44.73 0 bottom
C36  49.4,31.11 0 bottom
C37  49.63,48.13 180 bottom
C38  49.63,34.52 0 bottom
C39  49.63,41.33 180 bottom
C40  73.74,7.21 270 top
C41  74.04,82.23 180 bottom
C42  78.99,94.38 270 bottom
DRILEGEND  [DRILEGEND]  not placed on the board
FERRITE_BEAD  74.3,65.66 180 bottom
FTDI  64,95 180 top
IC1  69.52,74.08 90 top
J1  87.58,6.48 90 top
J2  84.45,95.63 0 top
LCDCONNECTOR  92.06,50.07 270 bottom
P1  33.19,39.5 180 top
PROXIMITYSENSOR  47,4 0 top
Q1  52.7,64.64 180 top
Q2  44.32,51.69 90 top
R1  81.28,61.98 270 bottom
R2  24.26,58.67 270 bottom
R3  55.01,67.37 0 top
R4  887k  [R0805']  69.15,27.79 180 bottom
R5  121k  [R0805']  80.44,26.8 270 bottom
R6  49.9k  [R0805']  67.64,18.92 270 bottom
R7  6.49k  [R0805']  72.15,24.89 180 bottom
R8  90.9k  [R0805']  79.45,16.89 0 bottom
R9  1k  [R0805']  79.45,21.34 180 bottom
R10  5k  [R0805']  64.9,23.62 90 top
S1  41.27,93.73 90 top
U1  60.2,39.88 0 top
U$1  65.93,6.99 90 top
U$2  56.34,20.07 0 top
X2  13.16,82.42 180 top

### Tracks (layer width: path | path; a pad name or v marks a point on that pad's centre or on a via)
1.8V  (via drill 0.33, 0.33 pad 0.55)
  Top 0.203: v53.59,36.58 55.44,36.58 U1.8
  Bottom 0.203: C36.1 50.58,31.32 C38.1 52.64,36.58 v53.59,36.58 53.59,33.92 C36.1
  other vias: 52.58,35.56 52.58,33.53
  pour Top: 53.34,37.59 56.39,37.59 56.39,36.07 53.85,36.07 53.85,33.53 52.32,32 52.32,29.46 43.43,29.46 43.43,35.81 51.56,35.81
  pour Bottom: 49.78,35.81 49.78,29.46 52.32,29.46 52.32,32 53.85,33.53 53.85,36.07 56.39,36.07 56.39,37.59 53.34,37.59 51.56,35.81
  pour Top (rank 2): 43.43,35.31 43.43,51.44 45.97,51.44 45.97,35.31
1.8V_MOSFET  (via drill 0.33)
  Top 0.203: IC1.2 61.27,62.07 61.35,61.99 61.35,60.85 v60.71,60.2 | v42.56,50.55 43.58,50.55 Q2.1
  Bottom 0.203: v60.71,60.2 60.71,54.74 59.18,53.21 45.23,53.21 v42.56,50.55
1.8V_PI  (via drill 0.33, 0.33 pad 0.55)
  Top 0.203: v32,63.75 v32,66.55 | v33.78,63.75 v33.78,66.55
  Bottom 0.203: v32,63.75 31.15,63.75 C31.1 C32.1 35.01,63.75 v33.78,63.75 | v39.62,62.74 C33.1
  other vias: 43.69,58.17 44.58,58.17 44.58,57.28 43.69,57.28 43.69,56.39 44.58,56.39
  pour Top: 27.69,67.06 35.31,67.06 35.56,66.8 38.86,66.8 38.86,66.04 30.73,66.04 30.48,66.29 27.69,66.29
  pour Top (rank 2): 43.18,59.56 43.18,51.94 45.97,51.94 45.97,59.56
  pour Bottom: 39.24,61.85 41.02,60.07 43.18,60.07 43.18,55.12 45.21,55.12 45.21,60.45 43.81,61.85
  pour Bottom: 23.75,63.5 43.05,63.5 43.18,63.37 43.18,61.47 23.24,61.47 23.24,63.5
5VIN  (via drill 0.33 pad 0.55)
  Top 0.203: J1.VIN0 78.56,6.48 76.44,8.6 C40.1 68.24,8.6 66.25,6.6 U$1.6
  Bottom 0.203: C22.1 50.79,41.12 C39.2 52.58,39.33 v52.58,39.12 51.38,37.92 C22.1
  pour Top (rank 2): 64.77,3.56 64.77,6.86 66.55,8.64 66.8,8.89 71.37,8.89 73.15,10.67 83.57,10.67 83.57,4.57 78.23,4.57 75.69,7.11 67.31,7.11 66.55,6.35 66.29,6.1 66.29,3.56
  pour Top: 78.49,14.99 78.49,4.57 83.57,4.57 83.57,12.83 58.42,37.97 58.42,39.88 49.53,39.88 49.53,36.32 51.31,36.32 53.59,38.61 56.9,38.61 56.9,36.58
5VOUT  (via drill 0.33, 0.33 pad 0.55)
  Top 0.203: C21.1 63.21,5.83 63.65,5.39 U$1.2 U$1.3 64.21,4.25 v64.21,5.59 | P1.200 25.27,71.15 23.61,69.49 16.11,69.49 9.66,75.94 X2.1
  Bottom 0.203: R7.1 71.1,24.89 R4.1 68.33,27.91 v68.33,31.24 | C29.1 C28.1 35.23,72.58 33.88,71.23 32.49,71.23 31.14,72.58 C27.1 C30.1
  other vias: 62.23,27.94 62.99,28.7 63.75,26.42 67.56,30.48 66.29,31.75 67.06,32.51 26.42,72.39 39.37,72.39
  pour Top: 27.69,71.88 30.23,71.88 30.73,71.37 38.86,71.37 38.86,70.1 30.48,70.1 30.23,70.36 27.69,70.36
  pour Top: 7.62,76.2 42.93,76.2 42.93,71.12 28.19,71.12 24.64,67.56 24.64,23.37 24.89,23.11 48.01,23.11 49.78,23.11 49.78,12.45 50.8,11.43 53.09,11.43 54.1,10.41 54.1,7.87 54.36,7.62 63.25,7.62 64.01,7.62 64.52,7.11 64.52,3.56 63.5,3.56 63.5,4.83 63.25,5.08 53.59,5.08 52.07,6.6 52.07,9.14 51.56,9.65 49.28,9.65 48.01,10.92 48.01,21.34 21.84,21.34 21.84,67.06 7.37,67.06 7.37,76.2
  pour Top: 48.01,23.11 48.01,28.96 62.23,28.96 62.99,29.72 65.28,27.43 66.04,26.67 66.04,25.91 50.04,25.91 49.78,25.91 49.78,23.11
  pour Top: 65.41,31.62 76.2,42.42 95.76,42.42 95.76,39.62 77.72,39.62 67.56,29.46
  pour Bottom: 62.74,29.21 67.06,33.53 69.34,31.24 64.01,25.91 61.21,25.91 61.21,28.96 62.23,28.96 62.48,28.96
  pour Bottom: 23.62,73.41 42.93,73.41 42.93,71.12 23.62,71.12 23.11,71.12 23.11,73.41
D_N
  Top 0.203: P1.167 39.19,61.25 39.5,61.56 42.55,61.56 43.06,62.07 43.06,76.69 42.93,76.82 12.67,76.82 12,77.49 12,79.66 X2.2
D_P
  Top 0.203: X2.3 14.16,78.65 14.62,78.19 43.45,78.19 44.56,77.09 44.56,61.93 43.03,60.39 39.44,60.39 39.19,60.65 P1.165
FT_PD  (via drill 0.33 pad 0.55)
  Top 0.203: v81.79,70.1 81.57,70.33 IC1.47
  Bottom 0.203: LCDCONNECTOR.8 88.12,56.55 88.12,58.7 81.79,65.04 v81.79,70.1
GND  (via drill 0.33, 0.33 pad 0.55)
  Top 0.203: v62.94,11.68 63,11.63 U$1.20 | v58.12,10.92 C21.2 55.11,8.6 v55.07,8.64 | C40.2 73.74,3.68 v73.61,3.56 90.36,3.56 J1.GND J1.P$4 93.28,15.38 v93.17,15.49 | v69.04,2.03 69.04,3.98 U$1.10 68.76,4.07 68.76,3.2 68.49,2.92 67.4,2.92 67,3.32 67,4.07 U$1.7 66.81,4.07 66.81,3.32 66.41,2.92 63.71,2.92 63.07,2.29 v62.94,2.29 | v68.83,67.69 68.27,67.13 IC1.16 | v75.31,69.72 75.31,69.34 78.83,65.83 IC1.38 | v75.31,73.28 76.26,72.33 IC1.51 81.34,72.33 81.79,71.88 v82.04,71.88 v83.06,71.88 83.82,71.12 v84.33,71.12 v85.34,70.1 v86.36,69.09 | v75.31,76.83 77.98,76.83 78.47,77.33 IC1.61 81.64,77.33 v82.04,77.72 v83.57,77.72 v85.09,77.72 v86.36,77.72 v87.88,77.72 | v74.99,80.46 74.99,81.98 73.27,83.7 IC1.83 73.22,84.86 73.22,85.68 73.05,85.86 67.99,85.86 67.81,85.68 67.81,84.86 IC1.94 67.77,83.61 v70.99,80.39 | v62.87,80.39 61.27,81.99 IC1.107 61.27,86.73 57.65,90.35 FTDI.1 | v62.61,78.36 61.34,78.36 60.34,77.36 60.31,77.33 IC1.120 57.64,77.33 57.02,76.71 57.02,73.27 57.92,72.37 58.74,72.37 IC1.130 61.02,72.33 62.99,74.3 v62.87,74.3 | v26.67,56.64 28.98,56.64 P1.152 | v26.16,70.36 26.57,69.95 P1.196 30.76,69.95 31.06,69.65 P1.195 | IC1.31 75.8,63.31 75.8,62.24 75.41,61.85 v74.93,61.85 | U$1.11 68.86,11.96 v69.85,12.95 | v68.2,53.09 68.22,53.1 C3.2 C4.2 76.18,53.1 v76.2,53.09 | P1.188 26.94,67.55 26.92,67.56 26.8,67.44 26.8,65.91 26.92,65.79 29.05,65.79 P1.182 | P1.181 38.65,65.45 39.37,66.17 39.37,67.06 39.18,67.25 P1.187
  Bottom 0.203: v62.94,2.29 v62.94,11.68 60.4,11.68 59.64,10.92 v58.12,10.92 | v73.61,3.56 70.56,3.56 v69.04,2.03 | R5.2 80.44,21.38 R9.2 R8.1 91.77,16.89 v93.17,15.49 93.17,38.48 | C36.2 48.02,33.86 C38.2 48.02,35.18 C22.2 48.02,40.66 C39.1 48.02,41.99 C35.2 48.02,47.47 C37.1 | C13.2 68.89,67.63 v68.83,67.69 | C11.2 75.31,69.28 v75.31,69.72 | C15.1 75.5,73.28 v75.31,73.28 | C5.1 76.14,76.83 v75.31,76.83 | C6.1 76.26,79.19 v74.99,80.46 C41.2 | C9.2 70.58,80.81 v70.99,80.39 | C17.2 66.56,80.76 v66.93,80.39 | C8.2 62.55,80.71 v62.87,80.39 | C10.2 62.08,78.36 v62.61,78.36 | C14.1 v62.86,74.29 | v62.86,74.29 v62.87,74.3 | v62.86,74.29 62.86,73.54 63.75,72.65 63.75,71.39 61.38,69.02 61.13,69.02 C7.1 | C33.2 C32.2 C31.2 C34.2 | C24.2 C23.2 C26.2 C25.2 | C30.2 C27.2 32.41,74.48 32.49,74.57 33.88,74.57 33.96,74.48 C28.2 C29.2 | R2.2 25.29,56.64 v26.67,56.64 | C42.2 79.19,93.23 81.42,93.23 J2.3 J2.5 | PROXIMITYSENSOR.1 55.07,8.26 v55.07,8.64 | 93.17,38.48 LCDCONNECTOR.19 | 93.17,38.48 93.17,38.64 LCDCONNECTOR.20 | C1.2 37.34,93.73 v37.21,93.85 | C16.2 84.26,80.46 v84.33,80.39
  other vias: 84.33,65.28 39.88,70.1 82.3,74.93 83.57,74.93 84.84,74.93 86.11,74.93 87.38,74.93 88.65,74.93 89.92,74.93 91.19,74.93 92.2,74.93 95.25,71.12 95.25,67.56 95.25,64.26 95.25,61.21 96.77,71.12 96.77,67.56 96.77,64.26 96.77,61.21 98.17,71.12 98.3,67.44 98.3,64.26 98.17,61.21 70.1,55.12 72.14,55.12 74.17,55.12 35.31,95.25 37.21,95.25 35.18,93.85 35.18,92.46 37.21,92.46 84.2,16.51 85.6,16.51 87,16.51 88.39,16.51 89.79,16.51 91.19,16.51 91.19,15.11 89.79,15.11 88.39,15.11 87,15.11 85.6,15.11 84.2,15.11 93.73,16.89 95.12,16.89 96.52,16.89 95.12,15.49 96.52,15.49 95.12,14.1 96.52,14.1 95.12,12.7 96.52,12.7 42.67,53.59 42.67,48.9 42.67,43.94 42.67,36.45 42.67,29.97 41.15,56.01 41.15,48.9 41.15,40.64 41.15,33.02 48.13,59.82 51.05,59.82 48.26,56.26 43.81,63.63 43.81,72.77 42.16,77.47 36.2,77.47 29.72,77.47 24.13,77.47 18.41,77.47
  pour Top (isolate 0.305, rank 5): 0,100 100,100 100,0 0,0
  pour Top: 29.21,19.81 37.34,19.81 37.34,7.37 29.46,7.37 29.21,7.37
  pour Top (rank 3): 23.88,61.72 43.18,61.72 43.18,23.62 23.88,23.62 23.62,23.88 23.62,61.47
  pour Bottom (isolate 0.254, rank 3): 0,0 0,100.08 100.08,100.08 100.08,0
N$1  (via drill 0.33 pad 0.55)
  Top 0.203: IC1.71 80.29,82.3 v84.33,82.3
  Bottom 0.203: v84.33,82.3 82.61,82.3 C16.1
N$2  (via drill 0.33)
  Top 0.203: v64.9,80.39 61.77,83.52 IC1.106
  Bottom 0.203: C17.1 64.66,80.63 v64.9,80.39
N$3
  Bottom 0.203: R7.2 75.32,24.89 C20.2
N$4  (via drill 0.33)
  Top 0.203: v68.15,11.94 68.2,11.88 U$1.12
  Bottom 0.203: v68.15,11.94 67.64,12.45 R6.2 68.47,17.14 C19.1
N$5
  Bottom 0.203: R6.1 68.72,20.95 C18.1
N$6  (via drill 0.33)
  Top 0.203: v74.63,23.88 v74.63,26.42 | v73.1,15.49 71.33,13.72 68.02,13.72 67.39,13.08 67.39,11.3 67.55,11.14 U$1.13
  Bottom 0.203: R5.1 C20.1 76.24,27.79 R4.2 73.26,27.79 v74.63,26.42 | v74.63,23.88 74.63,22.48 C18.2 C19.2 v73.1,15.5 v73.1,15.49
N$7
  Top 0.203: U$1.15 66.25,14.2 U$2.2
  pour Top (isolate 0.305, rank 2): 62.18,25.4 56.72,25.4 56.59,25.27 56.59,14.73 62.18,14.73
  pour Top (rank 2): 66.29,9.14 66.29,14.22 61.72,18.8 61.72,14.99 62.74,14.99 64.77,12.95 64.77,9.14
N$8
  Top 0.203: U$1.18 64.3,12.61 62.44,14.48 54.82,14.48 52.29,17 U$2.1
  pour Top (isolate 0.305, rank 3): 50.5,25.4 56.34,25.4 56.34,14.73 50.37,14.73 50.37,25.27
  pour Top: 63.5,12.19 63.5,8.89 64.52,8.89 64.52,12.7 62.74,14.48 56.39,14.48 56.13,14.73 56.13,14.99 50.55,14.99 50.55,12.95 62.74,12.95
N$9  (via drill 0.33)
  Top 0.203: v68.28,6.1 68.28,4.24 U$1.9
  Bottom 0.203: R8.2 78.5,16.51 68.28,6.28 v68.28,6.1
N$10  (via drill 0.33)
  Top 0.203: v67.26,6.1 67.26,5.59 67.55,5.3 U$1.8
  Bottom 0.203: R9.1 77.17,20 77.17,16.06 67.26,6.15 v67.26,6.1
OSC_IN
  Top 0.203: IC1.23 71.77,62.12 70.61,60.96 68.71,60.96 67.31,59.56 25MHZ_OSC.1 66.52,57.37 C3.1
OSC_OUT
  Top 0.203: IC1.24 72.27,62.1 73.41,60.96 75.56,60.96 76.96,59.56 25MHZ_OSC.2 77.88,57.25 C4.1
QIO0
  Top 0.203: LCDCONNECTOR.5 94.49,57.57 94.49,74.17 92.83,75.83 IC1.58
QIO1
  Top 0.203: IC1.59 93.85,76.33 96.01,74.17 96.01,56.39 94.87,55.24 94.74,55.12 92.96,55.12 92.2,55.88 92.2,57.66 90.9,58.96 LCDCONNECTOR.4
QIO2
  Top 0.203: LCDCONNECTOR.11 95.33,48.8 97.51,50.97 97.51,74.49 95.17,76.83 IC1.60
QIO3
  Top 0.203: IC1.63 81.53,78.33 81.66,78.45 95.93,78.45 99.02,75.36 99.02,50.38 96.17,47.54 92.05,47.54 LCDCONNECTOR.12
QSPI_CS  (via drill 0.33)
  Top 0.203: LCDCONNECTOR.6 83.31,56.42 79.03,60.7 79.03,64.83 74.08,69.78 70,69.78 68.43,68.2 v64.77,68.2 | IC1.112 60.75,81.33 64.74,77.34 v64.77,77.34
  Bottom 0.203: v64.77,77.34 v64.77,68.2
QSPICLK
  Top 0.203: IC1.48 82.83,70.83 87.12,66.53 87.12,62.23 89.15,60.2 92.2,60.2 93.33,59.07 LCDCONNECTOR.3
RESET  (via drill 0.33 pad 0.55)
  Top 0.203: IC1.25 72.8,63.37 72.8,64.18 71.62,65.36 v71.62,69.13 | J2.10 85.09,98.17 51.23,98.17 S1.3
  Bottom 0.203: J2.10 88,96.27 88.88,95.38 88.88,93.81 78.44,83.36 72.34,83.36 71.75,82.77 71.75,69.25 v71.62,69.13 | S1.3 42.16,91.85 42.16,93.66 C1.1
RUN  (via drill 0.33 pad 0.55)
  Top 0.203: P1.177 39.14,64.25 40,65.11 v40,66 | v51,70 51.82,69.18 51.82,68.07 52.58,67.31 53.94,67.31 R3.1
  Bottom 0.203: v51,70 51,69.11 47.89,66 v40,66
RUN_5V  (via drill 0.33)
  Top 0.203: IC1.3 61.77,47.07 v61.85,46.99 | R10.2 63.43,24.57 v63.37,24.51
  Bottom 0.203: v61.85,46.99 61.85,28.48 61.58,28.21 61.58,26.3 v63.37,24.51
RUN_5V_MODULE
  Top 0.203: R10.1 64.9,17.14 66.93,15.11 66.93,9.83 U$1.14
SENSOR_UART  (via drill 0.33 pad 0.55)
  Top 0.203: v64,60 65,60 67,62 69,62 69.27,62.27 IC1.18
  Bottom 0.203: PROXIMITYSENSOR.3 45.73,47.73 50,52 59.95,52 62.09,54.14 62.09,58.09 v64,60
SWCLK  (via drill 0.33 pad 0.55)
  Top 0.203: v57,83 57.17,82.83 IC1.109
  Bottom 0.203: J2.4 83.19,98.03 76.94,98.03 74.99,96.08 74.99,91.07 71.92,88 59,88 57,86 v57,83
SWDIO  (via drill 0.33 pad 0.55)
  Top 0.203: v62.22,86.47 62.26,86.47 62.27,86.47 IC1.105
  Bottom 0.203: J2.2 81.92,97 77,97 76,96 76,91 72.22,87.22 62.96,87.22 v62.22,86.47
SWO  (via drill 0.33 pad 0.55)
  Top 0.203: v57,71 57.17,70.83 IC1.133
  Bottom 0.203: J2.6 84.45,97.55 83.12,98.88 75.88,98.88 74,97 74,91 72,89 58,89 56,87 56,71 v57,71
UART5_RX  (via drill 0.33 pad 0.55)
  Top 0.203: P1.51 38.69,26.45 41.91,29.67 41.91,57.4 v45.97,61.47 | v54.86,70.61 54.86,77.72 56.47,79.33 IC1.116
  Bottom 0.203: v45.97,61.47 54.86,70.36 v54.86,70.61
UART5_TX  (via drill 0.33 pad 0.55)
  Top 0.203: IC1.113 54.86,80.83 v54.86,80.77 | P1.53 37.35,27.12 38.51,27.12 40.39,29 40.39,57.02 45.97,62.61 v45.97,64.01
  Bottom 0.203: v45.97,64.01 46.1,63.88 47.12,63.88 54.86,71.63 v54.86,80.77
USART1_RX
  Top 0.203: FTDI.4 63.77,93.5 IC1.102
USART1_TX
  Top 0.203: FTDI.5 67.81,92.81 64.27,89.27 IC1.101
USB_OTGID  (via drill 0.33)
  Top 0.203: v26.8,61.47 29.01,61.47 P1.168
  Bottom 0.203: R2.1 26.05,61.47 v26.8,61.47
VDD  (via drill 0.33, 0.33 pad 0.55)  (1 unrouted)
  Top 0.203: v52.83,44.7 52.83,43.05 | v70.74,67.69 68.77,65.72 IC1.17 | v72.77,67.44 75.27,64.94 IC1.30 | v75.31,71.5 76.32,70.49 76.32,69.09 79.09,66.33 IC1.39 | v75.31,75.06 77.54,72.83 IC1.52 84.65,72.83 90.17,67.31 90.17,64.66 LCDCONNECTOR.1 | v75.31,78.61 76.1,77.83 IC1.62 | v78.11,82.55 78.38,82.83 IC1.72 80.26,88.91 77.22,91.95 v77.22,95 | v73.03,80.39 72.77,80.65 IC1.84 | v68.96,80.39 67.27,82.08 IC1.95 | IC1.108 60.66,84.71 v58.8,84.71 58.8,85.2 55,89 55,95 57,97 60.73,97 FTDI.3 | v62.87,76.33 62.37,76.83 IC1.121 | v62.87,72.26 62.43,71.83 IC1.131 | v58.93,63.5 58.93,65.18 IC1.144 | 52.83,43.05 47.37,43.05 v46.99,42.67 | 52.83,43.05 54.1,41.78 U1.4
  Bottom 0.203: C37.2 50.58,44.94 C35.1 50.81,44.7 v52.83,44.7 | v70.74,67.69 70.79,67.64 C13.1 FERRITE_BEAD.1 73,67.21 v72.77,67.44 | C11.1 75.31,71.18 v75.31,71.5 | C15.2 75.63,75.06 v75.31,75.06 | C5.2 76.26,78.61 v75.31,78.61 | C6.2 78.11,81.21 v78.11,82.55 | C41.1 73.09,80.46 v73.03,80.39 | C9.1 68.68,80.67 v68.96,80.39 | v58.8,84.71 60.65,82.86 C8.1 61.02,82.23 61.59,81.67 61.59,80.7 62.58,79.71 63.55,79.71 v64.01,79.25 64.01,77.98 63.5,77.47 63.43,77.54 C10.1 62.21,76.33 v62.87,76.33 | C14.2 61.13,72.26 v62.87,72.26 | C7.2 61,65.57 v58.93,63.5 | C42.1 79.03,95.29 | 79.03,95.29 79.33,95 J2.1 | v77.22,95 78.74,95 79.03,95.29 | PROXIMITYSENSOR.2 48.27,28.42 46.3,30.39 46.3,41.1 46.99,41.78 v46.99,42.67 | v66.8,67.06 66.74,66.99 C12.1
  pour Top: 58.8,84.71 58.8,63.5 80.14,63.5 80.14,85.09 58.8,85.09
  pour Top (rank 2): 56.52,41.15 53.34,41.15 51.56,42.93 49.66,42.93 49.66,53.21 52.96,56.52 52.96,67.18 62.36,67.18 62.36,62.48 54.61,62.48 54.61,56.13 51.69,53.21 51.69,45.85 53.34,45.85 54.1,45.09 54.1,42.55 56.52,42.55
VDD_MOSFET  (via drill 0.33)
  Top 0.203: IC1.1 60.77,61.79 v60.71,61.72 | v54.86,64.01 54.85,63.99 Q1.1
  Bottom 0.203: v60.71,61.72 57.15,61.72 v54.86,64.01
VDD_PI  (via drill 0.33, 0.33 pad 0.55)
  Top 0.203: P1.193 39.41,69.05 v39.88,68.58 | P1.192 27.77,68.75 27.69,68.83 27.56,68.83 | v26.16,68.83 27.56,68.83 | 27.56,68.83 28.07,69.35 P1.194
  Bottom 0.203: C26.1 C25.1 40.83,67.63 v39.88,68.58 | C23.1 C24.1 24.96,67.63 v26.16,68.83
  other vias: 45.34,68.71 46.86,68.71 48.39,68.71 45.34,67.69 46.86,67.69 48.39,67.69
  pour Top: 27.43,68.58 35.81,68.58 36.07,68.33 38.86,68.33 38.86,69.09 30.99,69.09 30.73,69.34 27.43,69.34
  pour Top (rank 2): 44.58,69.47 49.53,69.47 52.45,66.55 52.45,63.37 50.55,63.37 50.55,66.29 49.91,66.93 44.58,66.93
  pour Bottom: 23.24,68.58 43.69,68.58 44.58,69.47 49.53,69.47 49.53,66.93 44.2,66.93 43.69,66.42 23.24,66.42
VDDA  (via drill 0.33)
  Top 0.203: v75.31,67.44 75.82,66.93 75.82,65.15 76.77,64.2 IC1.33 76.77,62.52 76.99,62.3 77.48,62.3 v77.72,62.05
  Bottom 0.203: v75.31,67.44 75.59,67.15 FERRITE_BEAD.2 | R1.1 79.61,62.98 78.74,62.1 77.77,62.1 v77.72,62.05
VREF  (via drill 0.33)
  Top 0.203: v76.45,61.85 76.27,62.03 IC1.32
  Bottom 0.203: R1.2 80.41,61.85 79.06,61.85 78.62,61.41 77.46,61.41 77.01,61.85 v76.45,61.85

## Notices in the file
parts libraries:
Wurth_Elektronik_Passive_rev18f: Copyright: Würth Elektronik
SparkFun-Connectors: Licensing: Creative Commons ShareAlike 4.0 International - https://creativecommons.org/licenses/by-sa/4.0
